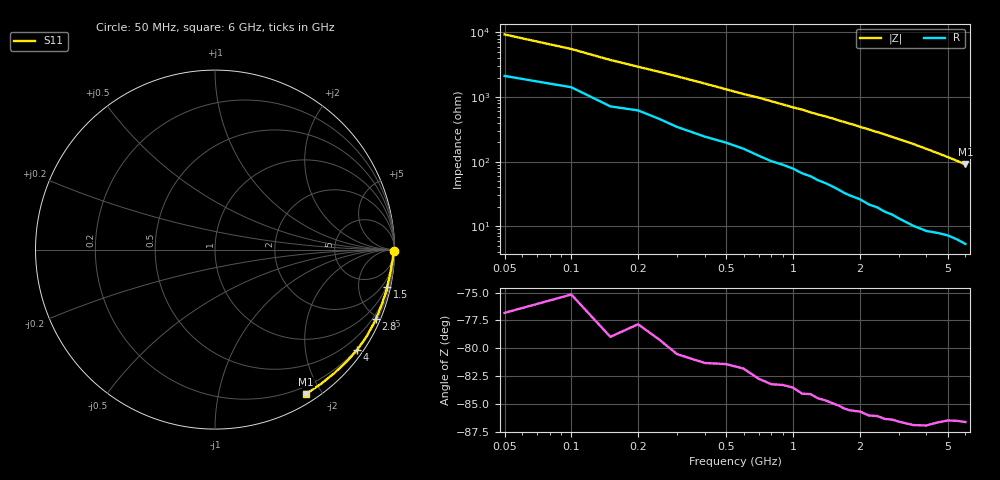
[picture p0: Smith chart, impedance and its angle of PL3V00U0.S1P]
! Infineon Technologies  Discrete & RF Semiconductors
! BAR 64-04W /-05W /-06W
! Si PIN Diode in SOT323
! VR = 3 V
! S-Parameters:  October  2008
# GHz  S  MA  R  50
!  f  S11
! GHz  MAG  ANG
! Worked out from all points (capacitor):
!   34 points, 50 MHz to 6 GHz, reference 50 ohm
!   read as one part to ground: C = 297 fF near 50 MHz
!   lowest |Z| = 90.5 ohm at 6 GHz (marker M1)
!   S11 on the Smith chart (normalised r, x): 50 MHz: open; 1.5 GHz: 0.83, -9.36; 2.8 GHz: 0.30, -4.83; 4 GHz: 0.17, -3.15; 6 GHz: 0.11, -1.81
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0.05  0.9976 -0.6
0.1  0.9954 -1.0
0.15  0.9949 -1.5
0.2  0.9929 -1.9
0.4  0.9907 -3.5
0.6  0.9873 -5.1
0.7  0.9872 -5.8
0.8  0.9864 -6.6
1  0.9839 -8.2
1.1  0.9841 -8.9
1.2  0.9826 -9.8
1.3  0.9825 -10.6
1.4  0.9819 -11.3
1.5  0.9815 -12.1
1.6  0.981 -13.0
1.7  0.981 -13.8
1.9  0.9799 -15.4
2.2  0.9788 -18.0
2.4  0.9772 -19.7
2.6  0.9769 -21.5
2.8  0.9754 -23.3
3  0.9749 -25.2
3.5  0.9733 -29.9
4  0.9696 -35.1
4.5  0.9628 -40.5
5  0.9569 -45.9
5.5  0.9534 -51.7
6  0.9513 -57.8
